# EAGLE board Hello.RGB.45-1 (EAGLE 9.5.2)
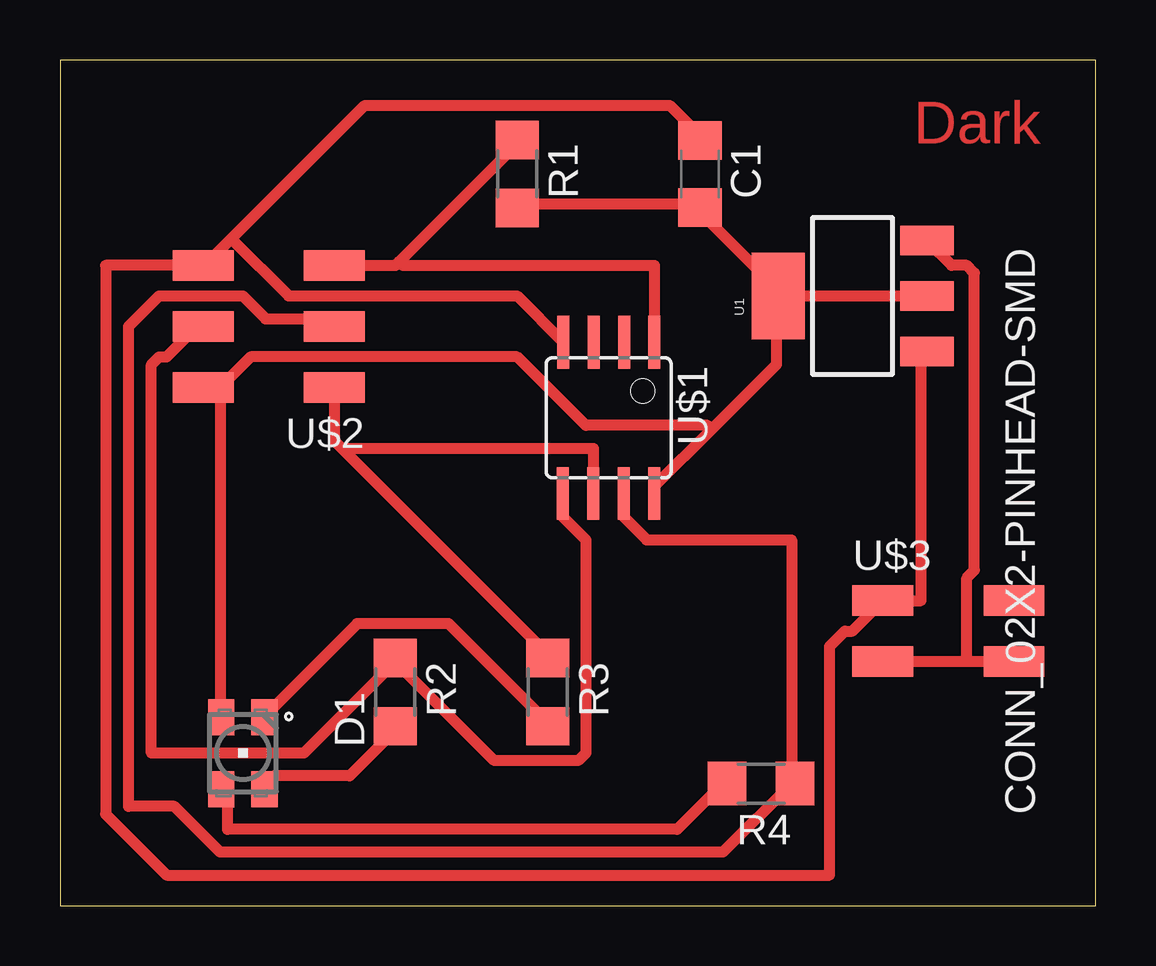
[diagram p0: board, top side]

Size 43.16 x 35.23 mm. Coordinates in mm from the lower left corner, seen from the top.
Outline: 0,0 43.16,0 43.16,35.23 0,35.23 0,0
Copper layers (1*16): Top 0.035mm / dielectric 1.5mm / Bottom 0.035mm
Design rules "fab-1": minimum track width 0.45mm, minimum drill 32mil, track to track 16mil, track to pad 16mil, pad to pad 16mil, via to via 16mil, smd to smd 6mil, copper to edge 16mil, drill to drill 16mil, minimum pad ring 10mil, minimum via ring 8mil, stop-mask expansion 4mil, vias tented up to drill 0mil, thermal gap 16mil

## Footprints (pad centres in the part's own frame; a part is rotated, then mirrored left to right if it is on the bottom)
C1206 = smd 1.6 x 1.8: 1 -1.4,0; 2 1.4,0
P-LCC-4 = smd 1.1 x 1.5: A 0.902,-1.5; B 0.902,1.5; G -0.902,1.5; R -0.902,-1.5
R1206 = smd 1.6 x 1.803: 1 -1.422,0; 2 1.422,0
SOT223 = smd 1.219 x 2.235: 1 -2.311,-3.099; 2 0,-3.099; 3 2.311,-3.099 | smd 3.6 x 2.2: 4 0,3.099
SOIC8 = smd 0.5 x 2.2: 1 -1.905,-3.154; 2 -0.645,-3.154; 3 0.625,-3.154; 4 1.895,-3.154; 5 1.905,3.154; 6 0.635,3.154; 7 -0.635,3.154; 8 -1.905,3.154
2X03SMD = smd 2.54 x 1.27: 1 -2.54,2.54; 2 2.92,2.54; 3 -2.54,0; 4 2.92,0; 5 -2.54,-2.54; 6 2.92,-2.54
2X02SMD = smd 2.54 x 1.27: 1 -2.54,1.27; 2 2.92,1.27; 3 -2.54,-1.27; 4 2.92,-1.27

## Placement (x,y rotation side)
C1  1UF  [C1206]  26.67,30.48 270 top
D1  LED_RGBNEW  [P-LCC-4]  7.62,6.35 180 top
R1  1Ok  [R1206]  19.05,30.48 270 top
R2  1K  [R1206]  13.97,8.89 270 top
R3  1K  [R1206]  20.32,8.89 270 top
R4  499  [R1206]  29.21,5.08 180 top
U1  VR_REGULATOR_SOT223  [SOT223]  33.02,25.4 90 top
U$1  UC_ATTINY45SI  [SOIC8]  22.86,20.32 180 top
U$2  CONN_03X2_AVRISPSMD  [2X03SMD]  8.89,24.13 180 top
U$3  CONN_02X2-PINHEAD-SMD  [2X02SMD]  36.83,11.43 0 top

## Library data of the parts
C1 D1 R1-R4 U1 U$1-U$3 = fab

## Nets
5V: U1.3 U$3.3 U$3.4
B: D1.B R4.2
G: D1.G R2.2
GND: C1.1 U1.1 U$1.4 U$2.6 U$3.1
MISO: R3.1 U$1.6 U$2.1
MOSI: R2.1 U$1.5 U$2.4
R: D1.R R3.2
RST: R1.1 U$1.1 U$2.5
SCK: R4.1 U$1.7 U$2.3
VCC: C1.2 D1.A R1.2 U1.2 U1.4 U$1.8 U$2.2

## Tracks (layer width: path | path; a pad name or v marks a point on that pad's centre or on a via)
5V
  Top 0.45: 37.78,10.16 37.78,13.65 38.1,13.97 38.1,26.35 37.78,26.67 37.15,26.67 36.19,27.62 U1.3 | U$3.4 37.78,10.16 | 37.78,10.16 U$3.3
B
  Top 0.45: D1.B 6.98,4.76 6.98,3.17 25.72,3.17 27.62,5.08 R4.2
G
  Top 0.45: D1.G 8.57,5.08 8.89,5.4 12.06,5.4 13.97,7.3 R2.2
GND
  Top 0.45: U1.1 35.88,22.86 35.88,12.7 U$3.1 33.02,11.43 32.7,11.43 32.07,10.79 32.07,1.27 4.44,1.27 1.9,3.81 1.9,26.67 U$2.6 6.03,26.67 7.14,27.78 | 7.14,27.78 12.7,33.34 25.4,33.34 26.67,32.07 C1.1 | 7.14,27.78 9.52,25.4 19.05,25.4 20.95,23.5 U$1.4
MISO
  Top 0.45: 11.91,18.89 11.43,19.37 U$2.1 | 11.91,18.89 20.32,10.48 R3.1 | U$1.6 22.22,19.05 12.06,19.05 11.91,18.89
MOSI
  Top 0.45: U$1.5 20.95,16.19 21.91,15.24 21.91,6.35 21.59,6.03 18.1,6.03 13.97,10.16 R2.1 13.97,9.84 13.65,9.84 10.16,6.35 3.81,6.35 3.81,22.54 4.13,22.86 4.44,22.86 5.71,24.13 U$2.4
R
  Top 0.45: D1.R 8.57,7.94 12.38,11.75 16.19,11.75 20.32,7.62 R3.2
RST
  Top 0.45: 14.13,26.83 13.97,26.67 U$2.5 | 14.13,26.83 19.05,31.75 R1.1 | U$1.1 24.76,26.67 14.29,26.67 14.13,26.83
SCK
  Top 0.45: 30.48,5.08 30.48,15.24 24.45,15.24 23.49,16.19 U$1.7 | U$2.3 11.11,24.45 8.57,24.45 7.62,25.4 4.13,25.4 2.86,24.13 2.86,4.13 4.76,4.13 6.67,2.22 27.62,2.22 30.48,5.08 | 30.48,5.08 R4.1
VCC
  Top 0.45: 6.67,21.59 6.67,7.94 D1.A | U$2.2 6.67,21.59 | 30.16,25.4 26.67,28.89 C1.2 26.67,29.21 19.05,29.21 R1.2 | 27.15,19.84 29.84,22.54 29.84,25.4 U1.4 30.16,25.4 | 27.15,19.84 24.76,17.46 U$1.8 | 30.16,25.4 U1.2 | 6.67,21.59 7.94,22.86 19.05,22.86 21.91,20 26.99,20 27.15,19.84

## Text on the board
Top: Dark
